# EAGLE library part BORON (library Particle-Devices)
BORON The Particle Boron cellular enabled development kit that can act as either a standalone cellular device or LTE enabled gateway, repeater, or endpoint for a Particle Mesh networks. More information: https://docs.particle.io/boron/ Footprint and formfactor based on Adafruit Feather.
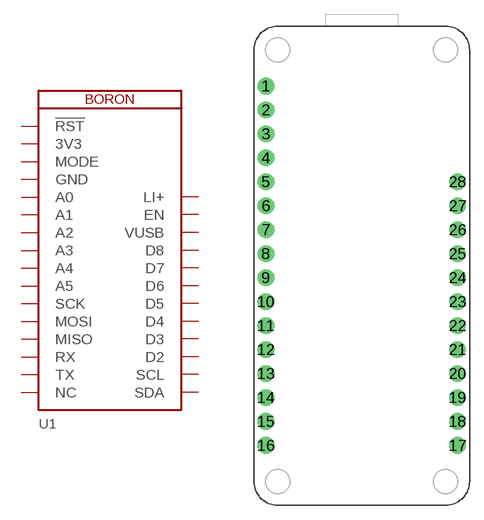
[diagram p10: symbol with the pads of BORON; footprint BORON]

Designator prefix U1

## BORON  [BORON]
1  !RST  in
2  3V3  pwr
3  MODE
4  GND  pwr
5  A0
6  A1
7  A2
8  A3
9  A4
10  A5
11  SCK
12  MOSI
13  MISO
14  RX
15  TX
16  NC
17  SDA
18  SCL
19  D2
20  D3
21  D4
22  D5
23  D6
24  D7
25  D8
26  VUSB  pwr
27  EN  in
28  LI+  pwr

## Footprint BORON (pad centres in mm)
BORON Footprint and formfactor based on Adafruit Feather. More information: https://docs.particle.io/boron/ Please pay attention to the keepout areas under the antenna to get good RF performance.
drill 1 pad 1.778: 1 1.27,44.45; 2 1.27,41.91; 3 1.27,39.37; 4 1.27,36.83; 5 1.27,34.29; 6 1.27,31.75; 7 1.27,29.21; 8 1.27,26.67; 9 1.27,24.13; 10 1.27,21.59; 11 1.27,19.05; 12 1.27,16.51; 13 1.27,13.97; 14 1.27,11.43; 15 1.27,8.89; 16 1.27,6.35; 17 21.59,6.35; 18 21.59,8.89; 19 21.59,11.43; 20 21.59,13.97; 21 21.59,16.51; 22 21.59,19.05; 23 21.59,21.59; 24 21.59,24.13; 25 21.59,26.67; 26 21.59,29.21; 27 21.59,31.75; 28 21.59,34.29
